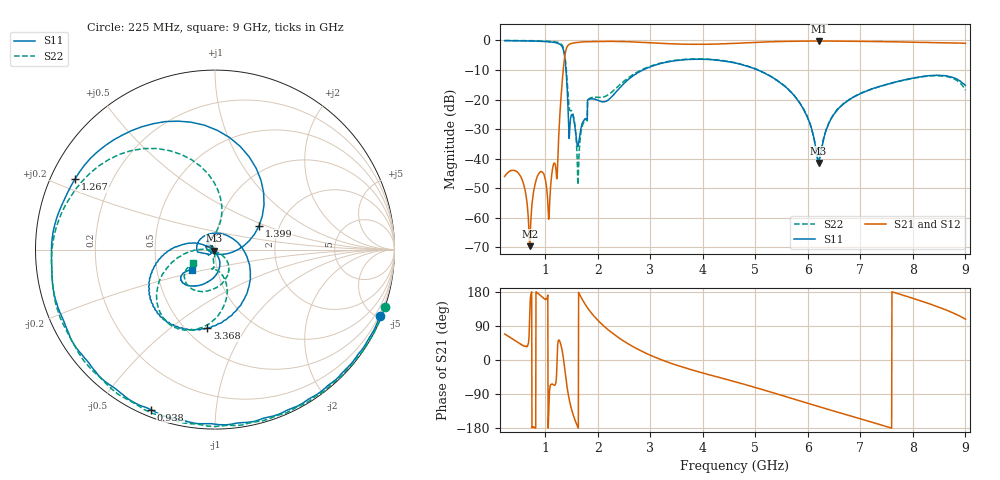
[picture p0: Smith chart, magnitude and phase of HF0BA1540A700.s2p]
!Agilent Technologies,E8358A,US41080443,A.07.50.56
!Agilent E8358A: A.07.50.56
!Date: Monday, March 28, 2016 12:52:01
!Correction: S11(Full 2 Port(1,2))
!S21(Full 2 Port(1,2))
!S12(Full 2 Port(1,2))
!S22(Full 2 Port(1,2))
!S2P File: Measurements: S11, S21, S12, S22:
# Hz S  dB  R 50
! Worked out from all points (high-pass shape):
!   1601 points, 225 MHz to 9 GHz, reference 50 ohm
!   highest |S21| = -0.18 dB at 6.214 GHz (marker M1); lowest = -69.6 dB at 702.1 MHz (marker M2)
!   |S21| within 3 dB of the highest: 1.394 GHz to end of sweep
!   lowest |S11| = -41.4 dB at 6.203 GHz (marker M3), VSWR 1.02, Z = 49.4 - j0.552 ohm
!   |S11| at or under -10 dB: 1.394 GHz to 2.86 GHz (1.466 GHz wide, 68.9 % of centre); 5.045 GHz to end of sweep
!   |S22| runs from -48.8 to 0.0 dB; largest |S21 - S12| = 0.014
!   S11 on the Smith chart (normalised r, x): 225 MHz: 0.10, -5.16; 938 MHz: 0.03, -0.68; 1.267 GHz: 0.07, +0.24; 1.399 GHz: 1.57, +0.45; 3.368 GHz: 0.63, -0.68; 9 GHz: 0.75, -0.18
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2.25e8  -0.06 -21.9  -46.04 68.4  -46.19 68.5  0.01 -18.5
5.266406e8  -0.11 -53.6  -45.92 42.3  -46.04 42.2  -0.03 -45.3
7.021406e8  -0.18 -75.2  -69.62 112.9  -69.29 112.8  -0.09 -63.5
9.379688e8  -0.35 -111.9  -44.47 166.2  -44.56 166.5  -0.18 -94.9
1.075078e9  -0.49 -140.3  -58.54 -96.7  -58.53 -94.7  -0.30 -119.2
1.267031e9  -1.17 153.4  -28.35 51.9  -28.47 52.0  -0.79 -175.9
1.398656e9  -11.08 28.5  -2.88 -55.0  -2.98 -54.9  -9.58 87.2
1.469953e9  -28.60 -171.7  -1.18 -113.5  -1.29 -113.4  -23.75 120.7
1.607062e9  -35.40 163.5  -0.65 -173.0  -0.75 -172.9  -40.13 135.1
1.689328e9  -28.80 -136.3  -0.52 163.4  -0.62 163.5  -30.15 -90.2
1.848375e9  -19.82 176.6  -0.43 129.2  -0.53 129.3  -19.57 -95.8
2.150016e9  -20.62 77.2  -0.32 85.2  -0.42 85.3  -18.86 -86.2
3.153656e9  -8.00 -82.3  -0.91 3.6  -1.02 3.7  -7.84 -93.2
3.367547e9  -7.17 -95.6  -1.11 -7.3  -1.21 -7.2  -7.03 -100.9
4.6125e9  -7.64 -151.8  -0.99 -57.3  -1.09 -57.2  -7.53 -140.6
5.566781e9  -15.58 168.7  -0.30 -96.1  -0.40 -96.0  -15.53 -172.5
6.076828e9  -30.27 160.0  -0.19 -117.4  -0.30 -117.4  -30.33 -177.6
6.202969e9  -41.43 -138.8  -0.19 -122.6  -0.29 -122.6  -41.78 -113.0
6.213938e9  -41.20 -119.5  -0.18 -123.2  -0.29 -123.1  -40.91 -94.0
6.581391e9  -23.18 -68.1  -0.25 -138.2  -0.36 -138.1  -23.06 -40.4
7.541156e9  -14.71 -102.8  -0.42 -177.5  -0.52 -177.4  -14.72 -75.0
9e9  -15.20 -138.8  -0.97 107.8  -1.06 108.0  -16.83 -149.6
